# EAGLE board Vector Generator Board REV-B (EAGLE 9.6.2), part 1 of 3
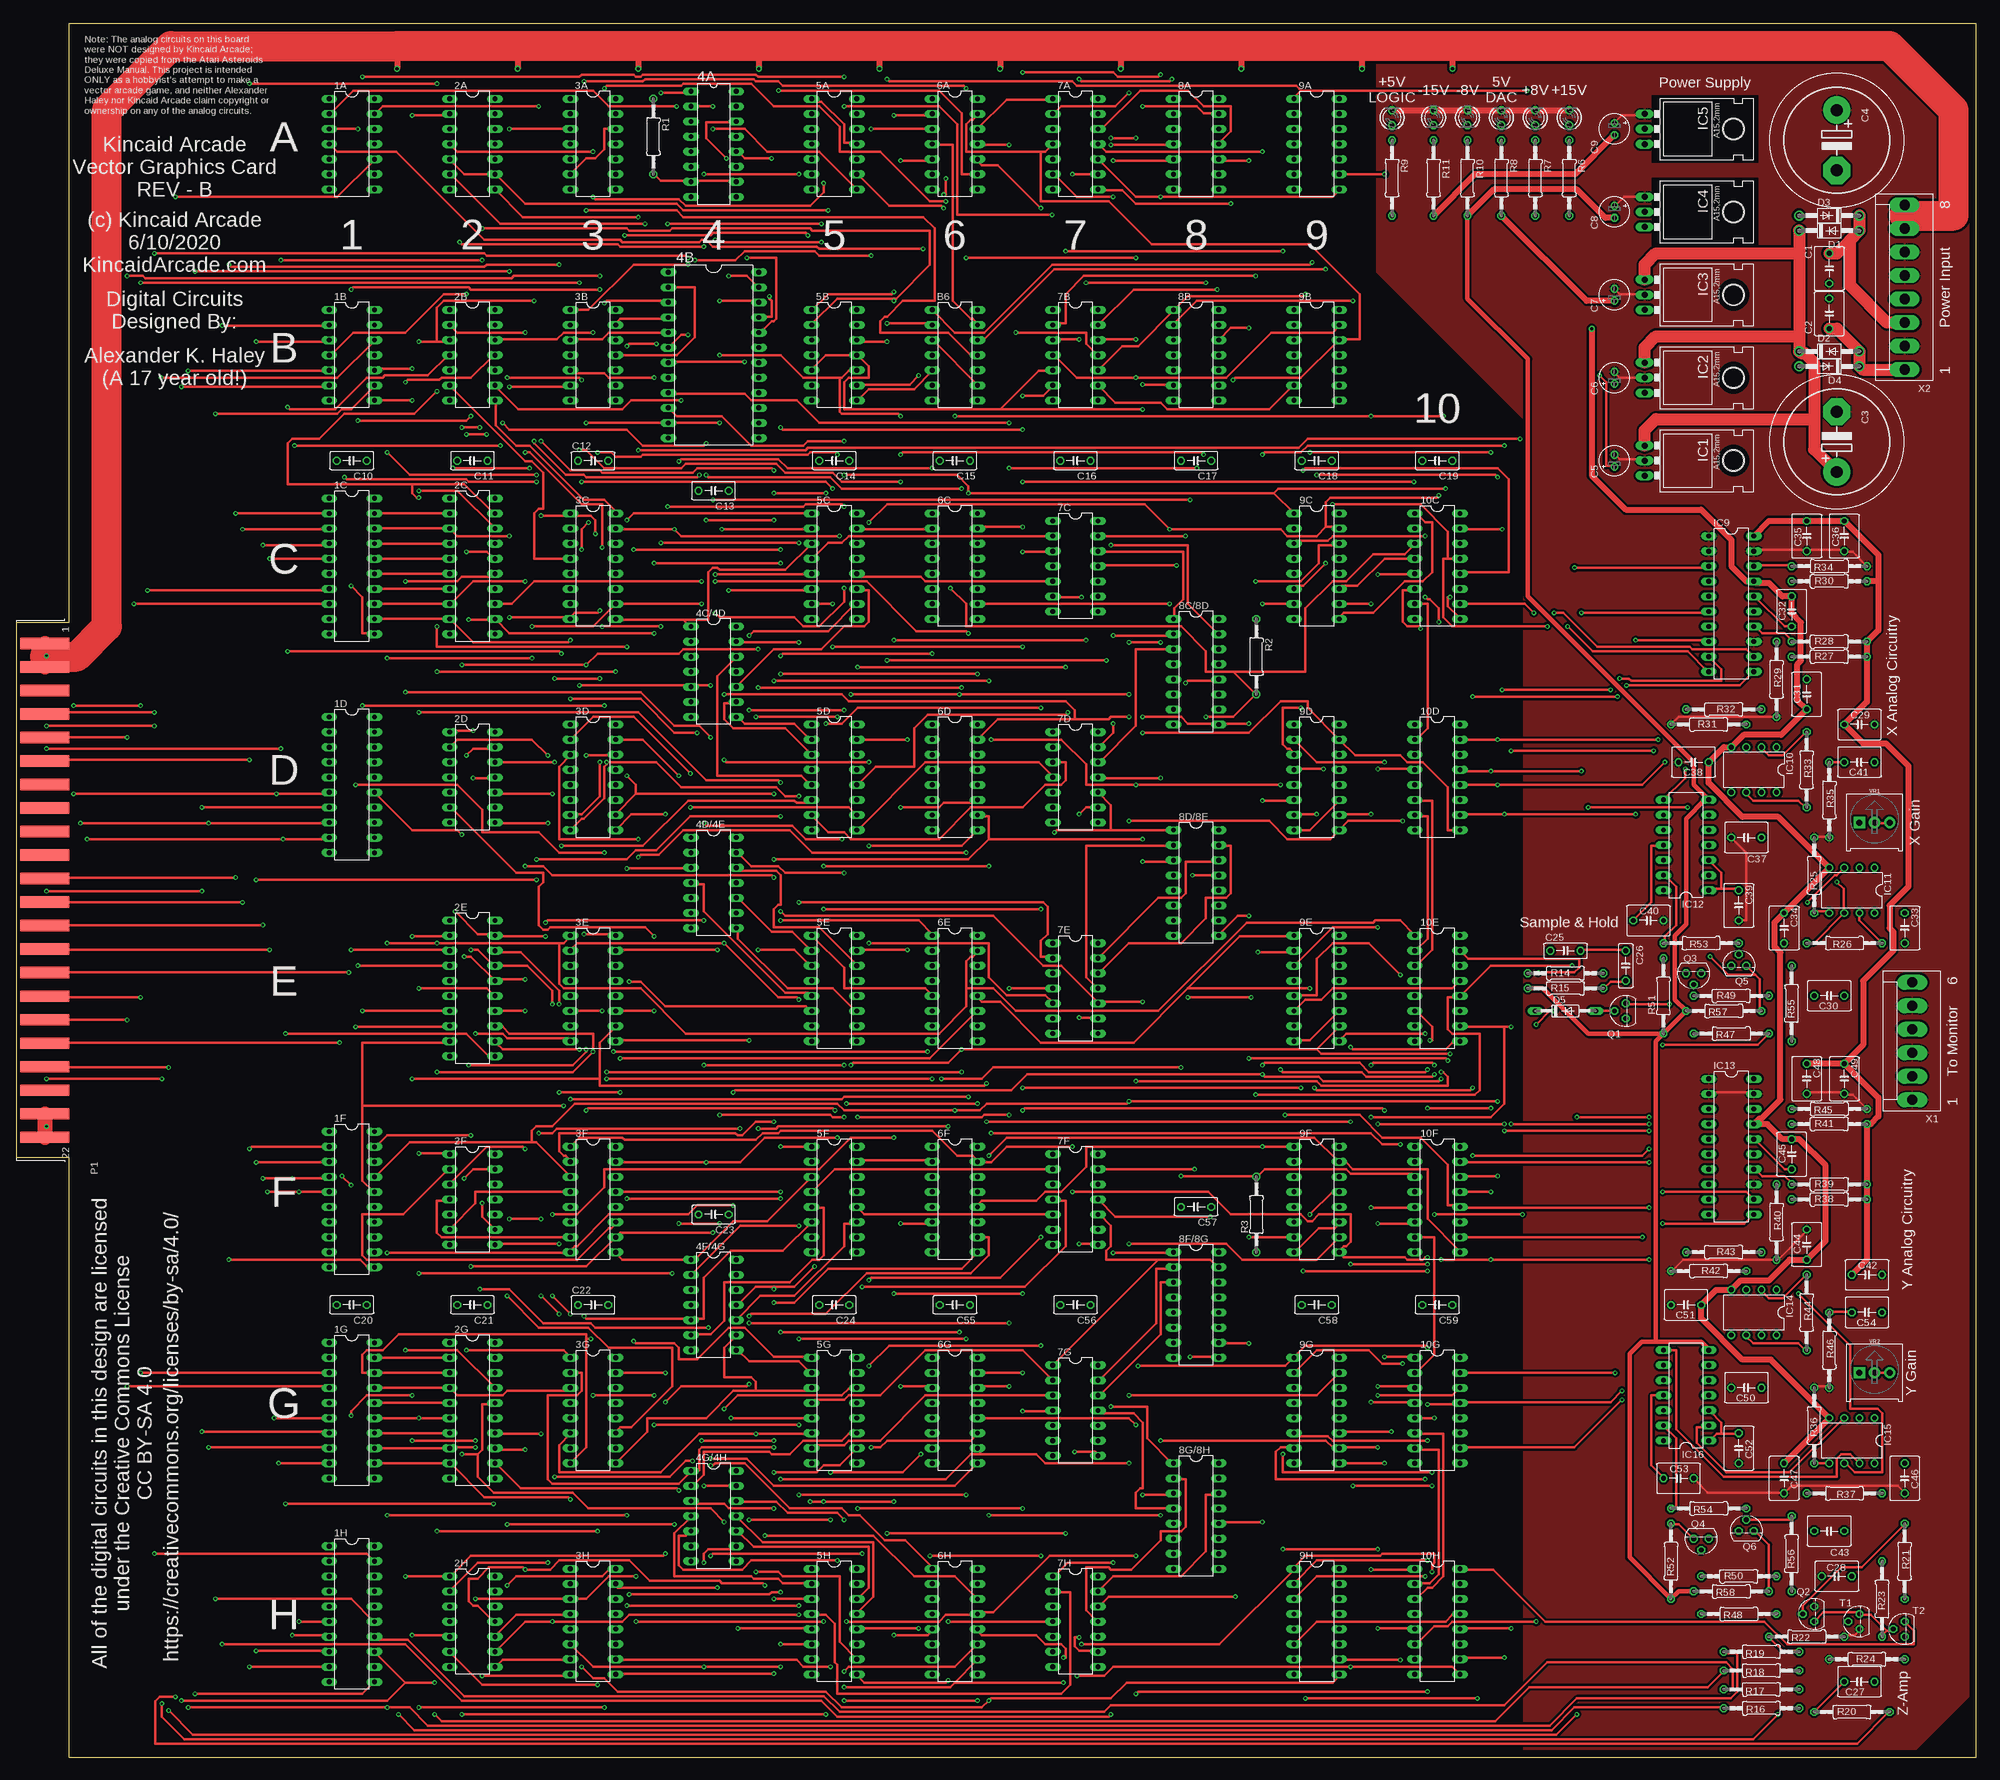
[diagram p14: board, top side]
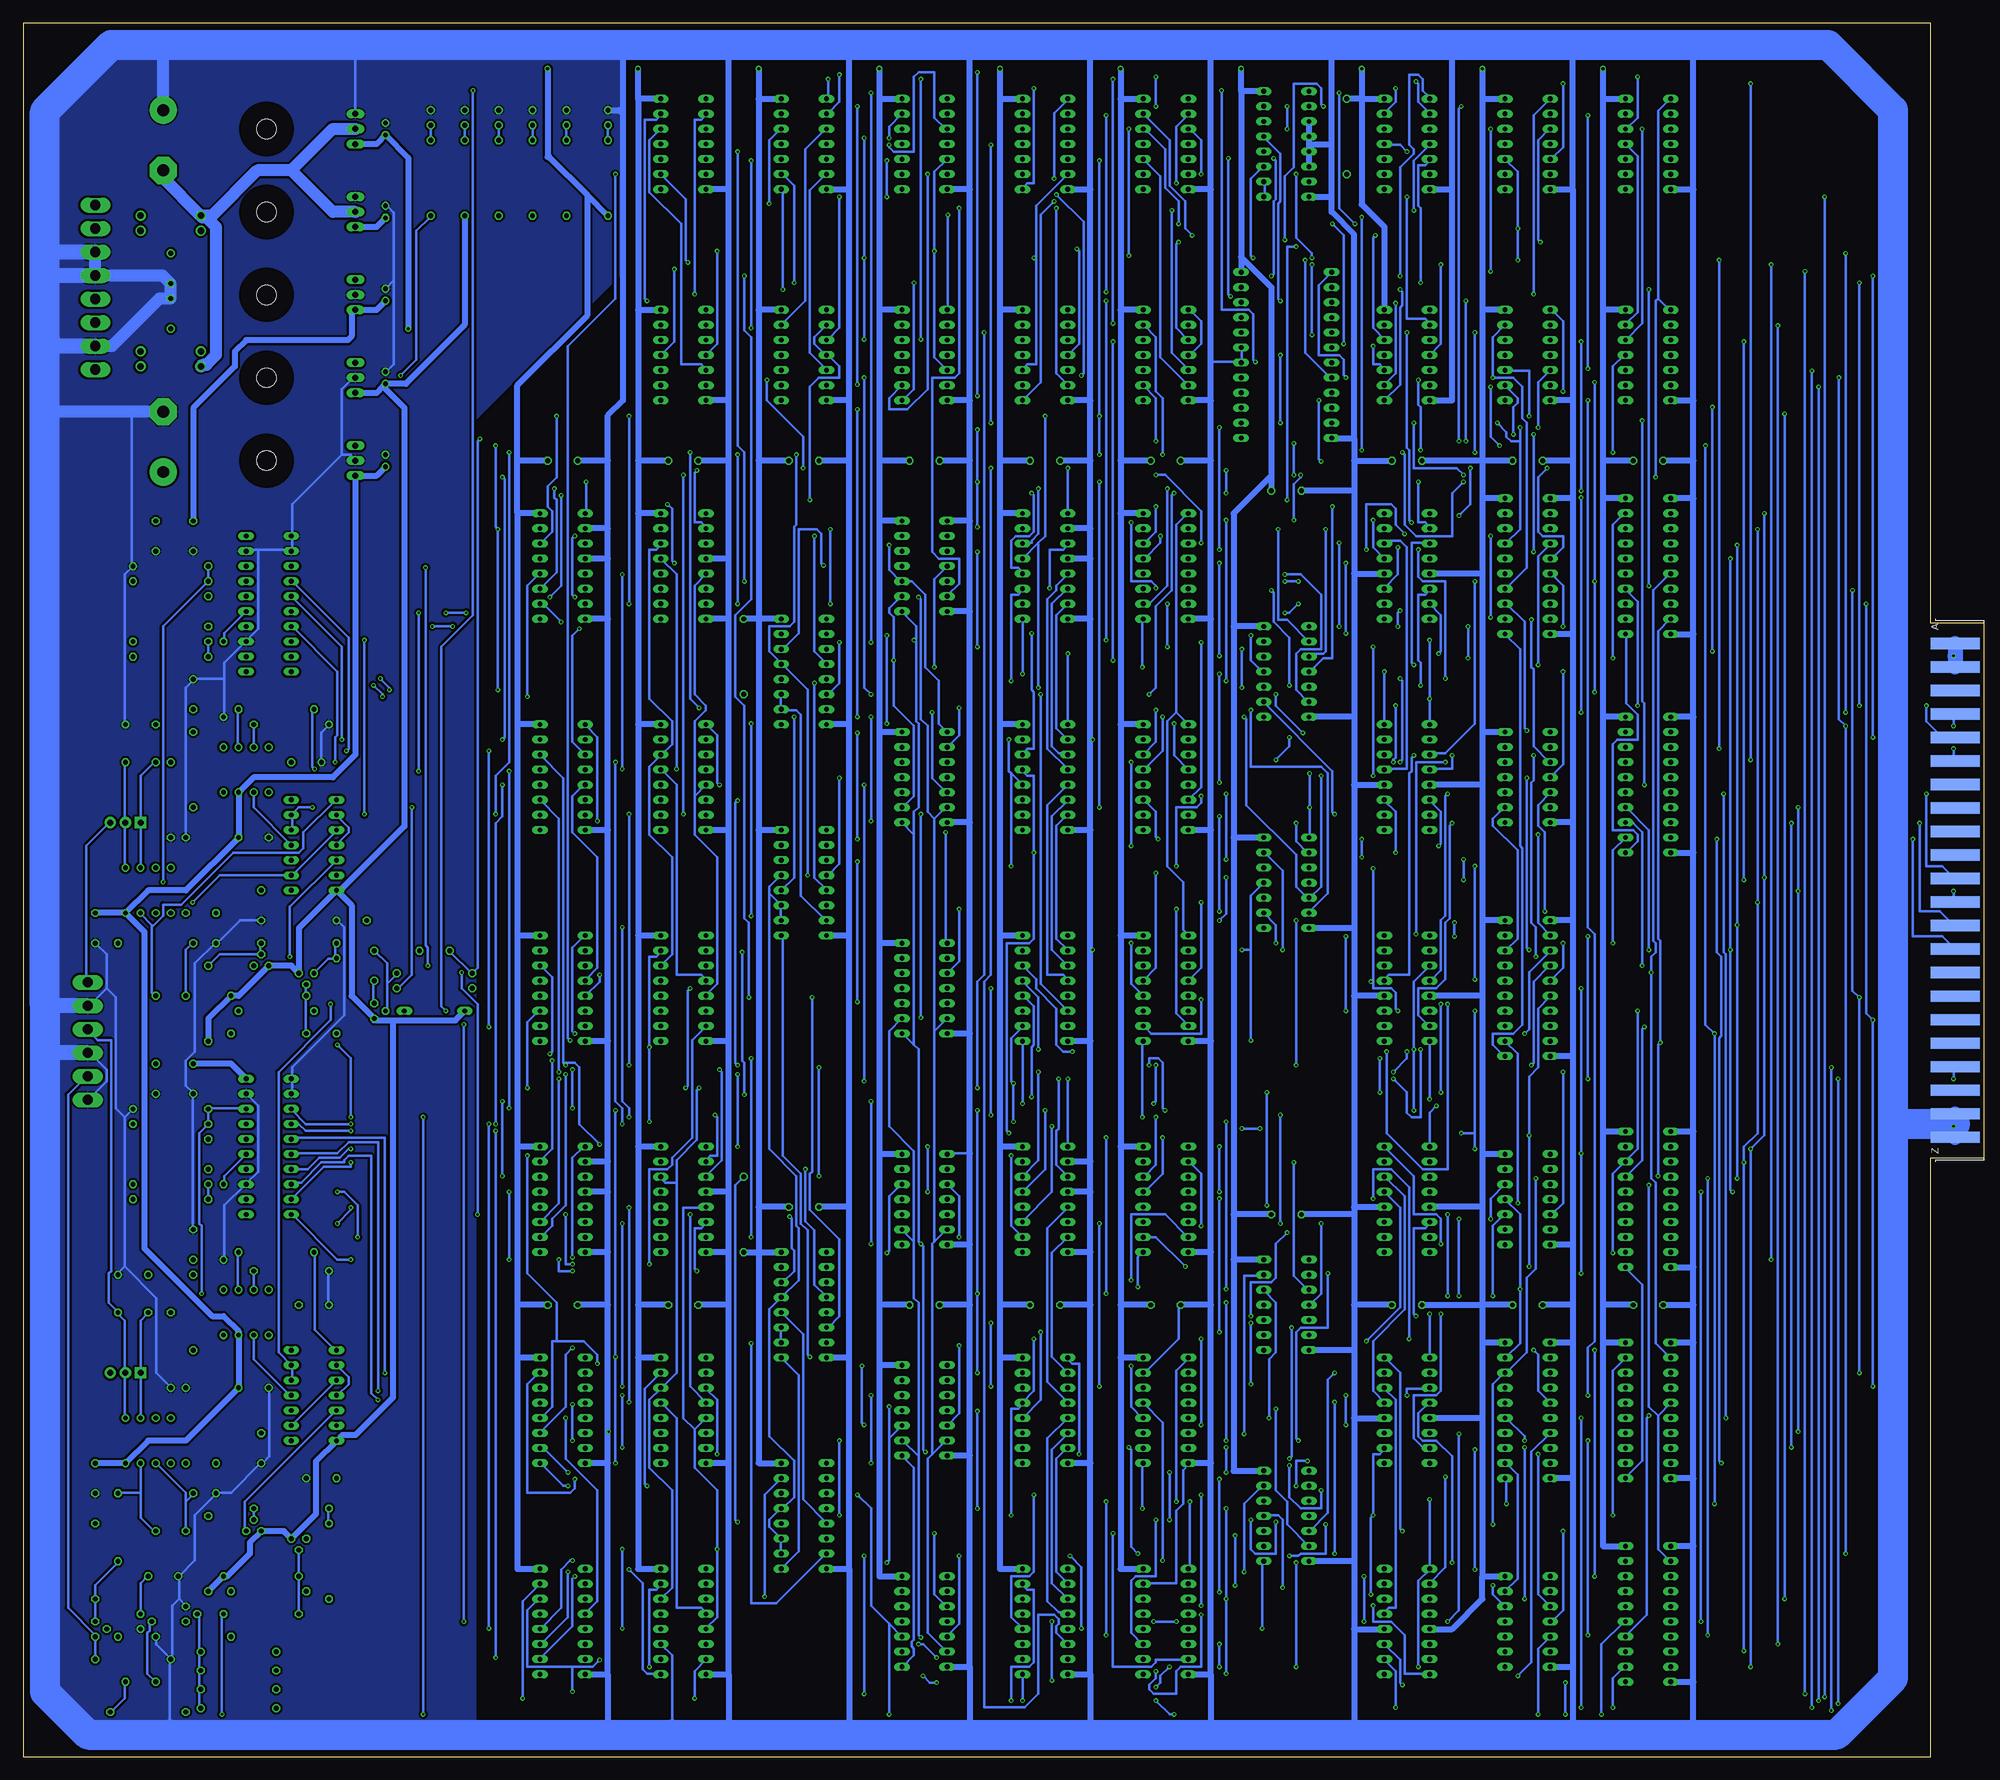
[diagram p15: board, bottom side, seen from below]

Size 330.2 x 292.1 mm. Coordinates in mm from the lower left corner, seen from the top.
Outline: 8.89,0 8.89,100.97 0,100.97 0,191.13 8.89,191.13 8.89,292.1 330.2,292.1 330.2,0 8.89,0
Copper layers (1*16): Top 0.035mm / dielectric 1.5mm / Bottom 0.035mm
Design rules "default": minimum track width 6mil, minimum drill 0.35mm, track to track 6mil, track to pad 6mil, pad to pad 6mil, via to via 6mil, smd to smd 6mil, copper to edge 40mil, drill to drill 6mil, minimum pad ring 10mil, minimum via ring 8mil, stop-mask expansion 4mil, vias tented up to drill 0mil, thermal gap 10mil
Net classes: 0 default: width 0.381 mm, clearance 0.381 mm

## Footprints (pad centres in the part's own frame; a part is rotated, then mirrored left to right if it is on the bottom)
DIL14 = drill 0.813 long: 1 -7.62,-3.81; 2 -5.08,-3.81; 3 -2.54,-3.81; 4 0,-3.81; 5 2.54,-3.81; 6 5.08,-3.81; 7 7.62,-3.81; 8 7.62,3.81; 9 5.08,3.81; 10 2.54,3.81; 11 0,3.81; 12 -2.54,3.81; 13 -5.08,3.81; 14 -7.62,3.81
DIL20 = drill 0.813 long: 1 -11.43,-3.81; 2 -8.89,-3.81; 3 -6.35,-3.81; 4 -3.81,-3.81; 5 -1.27,-3.81; 6 1.27,-3.81; 7 3.81,-3.81; 8 6.35,-3.81; 9 8.89,-3.81; 10 11.43,-3.81; 11 11.43,3.81; 12 8.89,3.81; 13 6.35,3.81; 14 3.81,3.81; 15 1.27,3.81; 16 -1.27,3.81; 17 -3.81,3.81; 18 -6.35,3.81; 19 -8.89,3.81; 20 -11.43,3.81
DIL16 = drill 0.813 long: 1 -8.89,-3.81; 2 -6.35,-3.81; 3 -3.81,-3.81; 4 -1.27,-3.81; 5 1.27,-3.81; 6 3.81,-3.81; 7 6.35,-3.81; 8 8.89,-3.81; 9 8.89,3.81; 10 6.35,3.81; 11 3.81,3.81; 12 1.27,3.81; 13 -1.27,3.81; 14 -3.81,3.81; 15 -6.35,3.81; 16 -8.89,3.81
DIL24-6 = drill 0.813 long: 1 -13.97,-7.62; 2 -11.43,-7.62; 3 -8.89,-7.62; 4 -6.35,-7.62; 5 -3.81,-7.62; 6 -1.27,-7.62; 7 1.27,-7.62; 8 3.81,-7.62; 9 6.35,-7.62; 10 8.89,-7.62; 11 11.43,-7.62; 12 13.97,-7.62; 13 13.97,7.62; 14 11.43,7.62; 15 8.89,7.62; 16 6.35,7.62; 17 3.81,7.62; 18 1.27,7.62; 19 -1.27,7.62; 20 -3.81,7.62; 21 -6.35,7.62; 22 -8.89,7.62; 23 -11.43,7.62; 24 -13.97,7.62
C050-050X075 = drill 0.813 octagon: 1 -2.54,0; 2 2.54,0
EB22,5D = drill 2.007 pad 4.597: + -5.08,0 | drill 2.007 pad 4.597 octagon: - 5.08,0
E2-5 = drill 0.813 pad 1.27: + -1.016,0 | drill 0.813 pad 1.27 octagon: - 1.016,0
C050-030X075 = drill 0.813 octagon: 1 -2.54,0; 2 2.54,0
C050-025X075 = drill 0.813 octagon: 1 -2.54,0; 2 2.54,0
DO41-10 = drill 1.118: A 5.08,0; C -5.08,0
DO35-10 = drill 0.813 long: A 5.08,0; C -5.08,0
78XXL = drill 1.016 long: GND 0,-3.81; IN -2.54,-3.81; OUT 2.54,-3.81 | hole 3.302: 0,11.176
79XXL = drill 1.016 long: GND -2.54,-3.81; IN 0,-3.81; OUT 2.54,-3.81 | hole 3.302: 0,11.176
DIL08 = drill 0.813 pad 1.27: 1 -3.81,-3.81; 2 -1.27,-3.81; 3 1.27,-3.81; 4 3.81,-3.81; 5 3.81,3.81; 6 1.27,3.81; 7 -1.27,3.81; 8 -3.81,3.81
LED3MM = drill 0.813 octagon: A -1.27,0; K 1.27,0
44PINEDGE = smd 1.905 x 8.255: 1 -41.605,4.826; 2 -37.643,4.826; 3 -33.68,4.826; 4 -29.718,4.826; 5 -25.756,4.826; 6 -21.793,4.826; 7 -17.831,4.826; 8 -13.868,4.826; 9 -9.906,4.826; 10 -5.944,4.826; 11 -1.981,4.826; 12 1.981,4.826; 13 5.944,4.826; 14 9.906,4.826; 15 13.868,4.826; 16 17.831,4.826; 17 21.793,4.826; 18 25.756,4.826; 19 29.718,4.826; 20 33.68,4.826; 21 37.643,4.826; 22 41.605,4.826 | smd 1.905 x 8.255 bottom: A -41.605,4.826; B -37.643,4.826; C -33.68,4.826; D -29.718,4.826; E -25.756,4.826; F -21.793,4.826; H -17.831,4.826; J -13.868,4.826; K -9.906,4.826; L -5.944,4.826; M -1.981,4.826; N 1.981,4.826; P 5.944,4.826; R 9.906,4.826; S 13.868,4.826; T 17.831,4.826; U 21.793,4.826; V 25.756,4.826; W 29.718,4.826; X 33.68,4.826; Y 37.643,4.826; Z 41.605,4.826
TO92 = drill 0.813 octagon: 1 1.27,0; 2 0,1.905; 3 -1.27,0
0207/12 = drill 0.813 octagon: 1 -6.35,0; 2 6.35,0
TRIMPOT-PTH-3386U = drill 1.016 pad 1.88 square: 1 -2.54,-0.015 | drill 1.016 pad 1.88: 2 0,-0.015; 3 2.54,-0.015
KK-156-6 = drill 1.7 pad 2.184 long: 1 -9.9,0; 2 -5.94,0; 3 -1.98,0; 4 1.98,0; 5 5.94,0; 6 9.9,0
KK-156-8 = drill 1.7 pad 2.184 long: 1 -13.86,0; 2 -9.9,0; 3 -5.94,0; 4 -1.98,0; 5 1.98,0; 6 5.94,0; 7 9.9,0; 8 13.86,0

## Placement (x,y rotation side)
1A  7404N  [DIL14]  56.52,271.78 270 top
1B  7402N  [DIL14]  56.52,236.22 270 top
1C  74HC573N  [DIL20]  56.52,200.66 270 top
1D  74HC573N  [DIL20]  56.52,163.83 270 top
1F  74HC573N  [DIL20]  56.52,93.98 270 top
1G  74HC573N  [DIL20]  56.52,58.42 270 top
1H  74HC573N  [DIL20]  56.52,24.13 270 top
2A  7400N  [DIL14]  76.84,271.78 270 top
2B  7404N  [DIL14]  76.84,236.22 270 top
2C  74HC573N  [DIL20]  76.84,200.66 270 top
2D  7404N  [DIL14]  76.84,165.1 270 top
2E  74HC573N  [DIL20]  76.84,129.54 270 top
2F  7404N  [DIL14]  76.84,93.98 270 top
2G  74HC573N  [DIL20]  76.84,58.42 270 top
2H  7404N  [DIL14]  76.84,22.86 270 top
3A  7432N  [DIL14]  97.16,271.78 270 top
3B  7404N  [DIL14]  97.16,236.22 270 top
3C  7483N  [DIL16]  97.16,200.66 270 top
3D  7483N  [DIL16]  97.16,165.1 270 top
3E  7483N  [DIL16]  97.16,129.54 270 top
3F  7483N  [DIL16]  97.16,93.98 270 top
3G  7483N  [DIL16]  97.16,58.42 270 top
3H  7483N  [DIL16]  97.16,22.86 270 top
4A  74161N  [DIL16]  117.48,271.78 270 top
4B  74154N  [DIL24-6]  117.48,236.22 270 top
4C/4D  7404N  [DIL14]  117.48,182.88 270 top
4D/4E  7404N  [DIL14]  117.48,147.32 270 top
4F/4G  7404N  [DIL14]  117.48,76.2 270 top
4G/4H  7404N  [DIL14]  117.48,40.64 270 top
5A  7432N  [DIL14]  137.8,271.78 270 top
5B  74S11N  [DIL14]  137.8,236.22 270 top
5C  74157N  [DIL16]  137.8,200.66 270 top
5D  74157N  [DIL16]  137.8,165.1 270 top
5E  74157N  [DIL16]  137.8,129.54 270 top
5F  74157N  [DIL16]  137.8,93.98 270 top
5G  74157N  [DIL16]  137.8,58.42 270 top
5H  74157N  [DIL16]  137.8,22.86 270 top
6A  7404N  [DIL14]  158.12,271.78 270 top
6C  7485N  [DIL16]  158.12,200.66 270 top
6D  7485N  [DIL16]  158.12,165.1 270 top
6E  7485N  [DIL16]  158.12,129.54 270 top
6F  7485N  [DIL16]  158.12,93.98 270 top
6G  7485N  [DIL16]  158.12,58.42 270 top
6H  7485N  [DIL16]  158.12,22.86 270 top
7A  74S08N  [DIL14]  178.44,271.78 270 top
7B  74S08N  [DIL14]  178.44,236.22 270 top
7C  7495N  [DIL14]  178.44,200.66 270 top
7D  7495N  [DIL14]  178.44,165.1 270 top
7E  7495N  [DIL14]  178.44,129.54 270 top
7F  7495N  [DIL14]  178.44,93.98 270 top
7G  7495N  [DIL14]  178.44,58.42 270 top
7H  7495N  [DIL14]  178.44,22.86 270 top
8A  7432N  [DIL14]  198.75,271.78 270 top
8B  74S11N  [DIL14]  198.75,236.22 270 top
8C/8D  7497N  [DIL16]  198.75,182.88 270 top
8D/8E  7497N  [DIL16]  198.75,147.32 270 top
8F/8G  7497N  [DIL16]  198.75,76.2 270 top
8G/8H  7497N  [DIL16]  198.75,40.64 270 top
9A  7404N  [DIL14]  219.07,271.78 270 top
9B  74S08N  [DIL14]  219.07,236.22 270 top
9C  74191N  [DIL16]  219.07,200.66 270 top
9D  74191N  [DIL16]  219.07,165.1 270 top
9E  74191N  [DIL16]  219.07,129.54 270 top
9F  74191N  [DIL16]  219.07,93.98 270 top
9G  74191N  [DIL16]  219.07,58.42 270 top
9H  74191N  [DIL16]  219.07,22.86 270 top
10C  7485N  [DIL16]  239.4,200.66 270 top
10D  7485N  [DIL16]  239.4,165.1 270 top
10E  7485N  [DIL16]  239.4,129.54 270 top
10F  7485N  [DIL16]  239.4,93.98 270 top
10G  7485N  [DIL16]  239.4,58.42 270 top
10H  7485N  [DIL16]  239.4,22.86 270 top
B6  74S08N  [DIL14]  158.12,236.22 270 top
C1  .1 uf  [C050-050X075]  305.44,250.82 270 top
C2  .1 uf  [C050-050X075]  305.44,243.21 90 top
C3  470 uf  [EB22,5D]  306.71,221.62 90 top
C4  470 uf  [EB22,5D]  306.71,272.41 270 top
C5  1 uf  [E2-5]  269.24,218.44 90 top
C6  1uf  [E2-5]  269.24,232.41 90 top
C7  1 uf  [E2-5]  269.24,246.38 90 top
C8  1uf  [E2-5]  269.24,260.35 270 top
C9  1 uf  [E2-5]  269.24,274.32 270 top
C10  .1uf  [C050-030X075]  56.52,218.44 180 top
C11  .1uf  [C050-030X075]  76.84,218.44 180 top
C12  .1uf  [C050-030X075]  97.16,218.44 0 top
C13  .1uf  [C050-030X075]  117.48,213.36 180 top
C14  .1uf  [C050-030X075]  137.8,218.44 180 top
C15  .1uf  [C050-030X075]  158.12,218.44 180 top
C16  .1uf  [C050-030X075]  178.44,218.44 180 top
C17  .1uf  [C050-030X075]  198.75,218.44 180 top
C18  .1uf  [C050-030X075]  219.07,218.44 180 top
C19  .1uf  [C050-030X075]  239.4,218.44 180 top
C20  .1uf  [C050-030X075]  56.52,76.2 180 top
C21  .1uf  [C050-030X075]  76.84,76.2 180 top
C22  .1uf  [C050-030X075]  97.16,76.2 0 top
C23  .1uf  [C050-030X075]  117.48,91.44 180 top
C24  .1uf  [C050-030X075]  137.8,76.2 180 top
C25  390pf  [C050-025X075]  260.99,135.89 0 top
C26  100pf  [C050-025X075]  271.14,133.35 270 top
C27  270pf  [C050-050X075]  310.51,12.7 180 top
C28  .01uf  [C050-050X075]  306.71,30.48 180 top
C29  .1uf  [C050-050X075]  310.51,173.99 0 top
C30  10pf  [C050-050X075]  305.44,128.27 180 top
C31  .1uf  [C050-050X075]  301.62,179.07 90 top
C32  .01uf  [C050-050X075]  299.09,193.04 90 top
C33  .1uf  [C050-050X075]  318.13,139.7 270 top
C34  .1uf  [C050-050X075]  297.81,139.7 270 top
C35  .1uf  [C050-050X075]  301.62,205.74 270 top
C36  .1uf  [C050-050X075]  307.98,205.74 270 top
C37  .1uf  [C050-050X075]  291.47,154.94 180 top
C38  .1uf  [C050-050X075]  282.58,167.64 180 top
C39  220pf  [C050-050X075]  290.19,143.51 270 top
C40  220pf  [C050-050X075]  274.96,140.97 0 top
C41  69pf  [C050-050X075]  310.51,167.64 180 top
C42  .1uf  [C050-050X075]  311.78,81.28 0 top
C43  10pf  [C050-050X075]  305.44,38.1 180 top
C44  .1uf  [C050-050X075]  301.62,86.36 90 top
C45  .01uf  [C050-050X075]  299.09,101.6 90 top
C46  .1uf  [C050-050X075]  318.13,46.99 270 top
C47  .1uf  [C050-050X075]  297.81,46.99 270 top
C48  .1uf  [C050-050X075]  301.62,114.3 270 top
C49  .1uf  [C050-050X075]  307.98,114.3 270 top
C50  .1uf  [C050-050X075]  291.47,62.23 180 top
C51  .1uf  [C050-050X075]  281.31,76.2 180 top
C52  220pf  [C050-050X075]  290.19,52.07 270 top
C53  220pf  [C050-050X075]  280.03,46.99 0 top
C54  69pf  [C050-050X075]  311.78,74.93 180 top
C55  .1uf  [C050-030X075]  158.12,76.2 180 top
C56  .1uf  [C050-030X075]  178.44,76.2 180 top
C57  .1uf  [C050-030X075]  198.75,92.71 180 top
C58  .1uf  [C050-030X075]  219.07,76.2 180 top
C59  .1uf  [C050-030X075]  239.4,76.2 180 top
D1  1N4004  [DO41-10]  305.44,257.18 0 top
D2  1N4004  [DO41-10]  305.44,236.85 0 top
D3  1N4004  [DO41-10]  305.44,259.72 180 top
D4  1N4004  [DO41-10]  305.44,234.31 180 top
D5  1N4148  [DO35-10]  260.99,125.73 0 top
IC1  7815  [78XXL]  278.13,218.44 270 top
IC2  7808  [78XXL]  278.13,232.41 270 top
IC3  7805  [78XXL]  278.13,246.38 270 top
IC4  7908  [79XXL]  278.13,260.35 270 top
IC5  7915  [79XXL]  278.13,274.32 270 top
IC9  DAC312  [DIL20]  288.93,194.31 270 top
IC10  TL081P  [DIL08]  292.74,166.37 180 top
IC11  TL082P  [DIL08]  309.25,146.05 180 top
IC12  4016N  [DIL14]  281.31,153.67 90 top
IC13  DAC312  [DIL20]  288.93,102.87 270 top
IC14  TL081P  [DIL08]  292.74,74.93 180 top
IC15  TL082P  [DIL08]  309.25,53.34 180 top
IC16  4016N  [DIL14]  281.31,60.96 90 top
LED1  [LED3MM]  261.62,276.23 90 top
LED2  [LED3MM]  255.91,276.23 90 top
LED3  [LED3MM]  250.19,276.23 90 top
LED4  [LED3MM]  231.78,276.23 90 top
LED5  [LED3MM]  244.47,276.23 270 top
LED6  [LED3MM]  238.76,276.23 270 top
P1  44PINEDGE  [44PINEDGE]  0,146.05 270 top
Q1  2N3906  [TO92]  271.14,125.73 90 top
Q2  2N3906  [TO92]  302.89,24.13 90 top
Q3  2N3906  [TO92]  282.58,132.08 180 top
Q4  2N3906  [TO92]  283.85,36.83 180 top
Q5  2N3906  [TO92]  290.19,133.35 0 top
Q6  2N3906  [TO92]  291.47,38.1 0 top
R1  1K  [0207/12]  107.32,273.05 270 top
R2  1K  [0207/12]  208.92,185.42 270 top
R3  1K  [0207/12]  208.92,91.44 90 top
R6  680  [0207/12]  261.62,266.06 270 top
R7  330  [0207/12]  255.91,266.06 270 top
R8  150  [0207/12]  250.19,266.06 270 top
R9  150  [0207/12]  231.78,266.06 270 top
R10  330  [0207/12]  244.47,266.06 270 top
R11  680  [0207/12]  238.76,266.06 270 top
R14  47K  [0207/12]  260.99,132.08 0 top
R15  330  [0207/12]  260.99,129.54 0 top
R16  1.2K  [0207/12]  294,8.26 0 top
R17  2.2K  [0207/12]  294,11.43 0 top
R18  4.7K  [0207/12]  294,14.61 0 top
R19  10K  [0207/12]  294,17.78 0 top
R20  1K  [0207/12]  309.25,7.62 0 top
R21  3.9K  [0207/12]  318.13,33.02 270 top
R22  22K  [0207/12]  301.62,20.32 180 top
R23  68  [0207/12]  314.33,26.67 90 top
R24  27  [0207/12]  311.78,16.51 0 top
R25  6.8K  [0207/12]  302.89,148.59 270 top
R26  8.2K  [0207/12]  307.98,137.16 180 top
R27  10k  [0207/12]  305.44,185.42 0 top
R28  10k  [0207/12]  305.44,187.96 0 top
R29  4.7K  [0207/12]  296.55,181.61 270 top
R30  10K  [0207/12]  305.44,198.12 0 top
R31  4.7K  [0207/12]  285.12,173.99 0 top
R32  10K  [0207/12]  287.65,176.53 0 top
R33  10K  [0207/12]  301.62,166.37 270 top
R34  2.2K  [0207/12]  305.44,200.66 180 top
R35  3.9K  [0207/12]  305.44,161.29 270 top
R36  6.8K  [0207/12]  302.89,55.88 270 top
R37  8.2K  [0207/12]  307.98,44.45 180 top
R38  10k  [0207/12]  305.44,93.98 0 top
R39  10k  [0207/12]  305.44,96.52 0 top
R40  4.7K  [0207/12]  296.55,90.17 270 top
R41  10K  [0207/12]  305.44,106.68 0 top
R42  4.7K  [0207/12]  285.12,81.91 0 top
R43  10K  [0207/12]  287.65,85.09 0 top
R44  10K  [0207/12]  301.62,74.93 270 top
R45  2.2K  [0207/12]  305.44,109.22 180 top
R46  3.9K  [0207/12]  305.44,68.58 270 top
R47  18K  [0207/12]  288.93,121.92 180 top
R48  18K  [0207/12]  290.19,24.13 180 top
R49  2.2K  [0207/12]  288.93,128.27 0 top
R50  2.2K  [0207/12]  290.19,30.48 0 top
R51  3.3K  [0207/12]  277.5,128.27 90 top
R52  3.3K  [0207/12]  278.76,33.02 90 top
R53  100K  [0207/12]  283.85,137.16 180 top
R54  100K  [0207/12]  285.12,41.91 180 top
R55  4.7K  [0207/12]  299.09,127 90 top
R56  4.7K  [0207/12]  299.09,34.29 90 top
R57  56K  [0207/12]  287.65,125.73 180 top
R58  56K  [0207/12]  288.93,27.94 180 top
T1  2N3904  [TO92]  310.51,22.86 90 top
T2  2N3904  [TO92]  318.13,21.59 90 top
VR1  10k  [TRIMPOT-PTH-3386U]  313.06,157.48 0 top
VR2  10k  [TRIMPOT-PTH-3386U]  313.06,64.77 0 top
X1  [KK-156-6]  319.4,120.65 90 top
X2  [KK-156-8]  318.13,247.65 90 top

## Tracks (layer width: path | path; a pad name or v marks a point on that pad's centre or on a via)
1DX0
  Top 0.381: 112.4,191.64 113.54,190.5 4C/4D.1 | 112.4,191.64 100.97,191.64 3C.9 | 5C.3 129.54,200.03 118.49,200.03 118.11,200.41 117.35,200.41 116.59,199.64 116.59,191.64 112.4,191.64
1DX1  (via drill 0.35)
  Top 0.381: v94.87,180.59 113.54,180.59 4C/4D.5 113.92,180.59 v116.97,180.59 | v120.02,196.6 133.73,196.6 5C.6
  Bottom 0.381: v94.87,180.59 94.87,184.4 95.25,184.78 95.25,195.83 94.11,195.83 93.34,196.6 3C.6 | v120.02,196.6 119.63,196.22 119.63,191.26 116.97,188.59 v116.97,180.59
1DX2  (via drill 0.35)
  Top 0.381: v95.25,214.88 136.4,214.88 v137.54,213.74 | v123.44,188.98 124.21,189.74 136.78,189.74 141.35,194.31 5C.10
  Bottom 0.381: v95.25,214.88 95.25,208.03 94.11,208.03 93.34,207.26 3C.2 | v137.54,213.74 137.54,197.36 140.59,194.31 5C.10 | v123.44,188.98 123.44,184.78 121.54,182.88 4C/4D.11
1DX3  (via drill 0.35)
  Top 0.381: 3C.15 100.97,206.88 v110.87,206.88 112.01,205.74 v138.68,205.74
  Bottom 0.381: v110.87,206.88 110.87,186.31 111.25,185.93 113.54,185.93 113.54,185.55 4C/4D.3 | v138.68,205.74 138.68,204.6 141.35,201.93 5C.13
1DX4  (via drill 0.35)
  Top 0.381: 3D.9 103.63,158.88 v109.35,158.88 | 5D.3 129.54,173.36 120.78,173.36 119.25,174.88 119.25,177.55 121.16,177.55 4C/4D.9
  Bottom 0.381: v109.35,158.88 109.73,159.26 109.73,166.12 121.16,177.55 4C/4D.9
1DX5  (via drill 0.35)
  Top 0.381: v91.82,153.54 105.54,153.54 113.16,161.16 131.06,161.16 131.44,160.78 133.35,160.78 133.73,161.16 5D.6 | v131.83,187.83 121.54,187.83 4C/4D.13
  Bottom 0.381: v91.82,153.54 91.44,153.92 91.44,159.26 93.34,161.16 3D.6 | v131.83,187.83 131.83,163.45 5D.6
1DX6  (via drill 0.35)
  Top 0.381: 3D.2 97.16,175.26 104.01,175.26 v113.54,165.74 | v113.54,160.02 140.21,160.02 141.35,158.88 5D.10
  Bottom 0.381: v113.54,165.74 v113.54,160.02 113.54,155.07 4D/4E.1
1DX7  (via drill 0.35)
  Top 0.381: v111.63,165.35 105.54,171.45 3D.15 | v124.59,175.26 v138.3,175.26
  Bottom 0.381: v111.63,165.35 111.63,146.69 113.54,144.78 4D/4E.5 113.92,144.78 115.82,146.69 115.82,152.02 124.21,160.4 124.21,174.88 v124.59,175.26 | v138.3,175.26 138.3,169.55 141.35,166.5 5D.13
1DX8  (via drill 0.35)
  Top 0.381: v123.44,120.78 100.97,120.78 3E.9 | v124.97,136.02 131.06,136.02 133.73,133.35 5E.3
  Bottom 0.381: 123.44,136.02 123.44,145.16 4D/4E.11 | 123.44,136.02 v123.44,120.78 | 123.44,136.02 v124.97,136.02
1DX9  (via drill 0.35)
  Top 0.381: v98.68,125.73 3E.6 | v102.87,149.73 113.54,149.73 4D/4E.3 | v103.25,130.68 105.16,130.68 109.35,126.49 132.97,126.49 133.73,125.73 5E.6
  Bottom 0.381: v98.68,125.73 99.06,126.11 99.06,128.78 99.82,129.54 102.87,129.54 102.87,130.68 | v102.87,149.73 102.87,130.68 | 102.87,130.68 v103.25,130.68
1DX10  (via drill 0.35)
  Top 0.381: 3E.2 93.34,136.02 94.49,137.16 v119.25,137.16 128.4,128.02 131.44,128.02 v131.83,127.64
  Bottom 0.381: v119.25,137.16 119.25,140.21 4D/4E.9 | v131.83,127.64 131.83,121.92 140.21,121.92 141.35,123.06 5E.10
1DX11  (via drill 0.35)
  Top 0.381: v118.11,136.02 100.97,136.02 3E.15 | v139.45,148.97 129.54,148.97 128.4,150.11 123.83,150.11 121.54,152.4 4D/4E.13
  Bottom 0.381: v118.11,136.02 118.11,149.35 121.16,152.4 4D/4E.13 | 5E.13 139.45,132.97 v139.45,148.97
1DY0
  Top 0.381: 3F.9 100.97,84.96 102.11,83.82 4F/4G.1 114.3,83.82 120.78,90.3 126.49,90.3 5F.3
1DY1  (via drill 0.35)
  Top 0.381: v95.63,74.3 96.01,73.91 113.54,73.91 4F/4G.5 113.92,73.91 115.82,73.91 115.82,80.77 120.4,85.34 129.16,85.34 5F.6
  Bottom 0.381: v95.63,74.3 96.01,74.68 96.01,89.15 94.11,89.15 93.34,89.92 3F.6
1DY2  (via drill 0.35)
  Top 0.381: 127.64,79.25 131.06,79.25 v134.49,82.68 | 127.64,79.25 124.59,79.25 121.54,76.2 4F/4G.11 | v127.64,107.06 124.59,107.06 122.3,104.78 121.54,104.78 121.16,105.16 91.44,105.16 91.44,102.11 92.2,101.35 92.58,101.35 93.34,100.58 3F.2 | 127.64,79.25 v127.64,78.87
  Bottom 0.381: v134.49,82.68 139.45,87.63 5F.10 | v127.64,78.87 v127.64,107.06
1DY3  (via drill 0.35)
  Top 0.381: 3F.15 100.97,100.2 v116.21,100.2 121.92,100.2 126.11,104.39 v138.3,104.39
  Bottom 0.381: v116.21,100.2 116.21,81.15 113.92,78.87 4F/4G.3 | v138.3,104.39 138.3,98.3 141.35,95.25 5F.13
1DY4
  Top 0.381: 3G.9 106.3,54.86 106.3,57.15 116.21,57.15 120.78,61.72 124.59,61.72 | 124.59,61.72 133.35,61.72 133.73,62.1 5G.3 | 124.59,61.72 124.59,63.25 123.83,64.01 119.25,64.01 119.25,68.96 121.16,70.87 4F/4G.9
1DY5  (via drill 0.35)
  Top 0.381: 3G.6 93.34,54.48 91.44,52.58 91.44,48.01 108.59,48.01 115.06,54.48 v124.59,54.48 133.73,54.48 5G.6
  Bottom 0.381: v124.59,54.48 124.59,81.15 121.54,81.15 4F/4G.13
1DY6  (via drill 0.35)
  Top 0.381: 3G.2 95.25,64.77 95.25,61.72 94.49,60.96 89.54,60.96 89.54,46.86 90.3,46.1 111.63,46.1 113.54,48.01 4G/4H.1 113.92,48.39 115.06,48.39 115.06,51.82 115.44,52.2 v127.64,52.2 | 5G.10 138.68,49.15 136.02,49.15 134.87,48.01 v127.64,48.01
  Bottom 0.381: v127.64,52.2 v127.64,48.01
1DY7  (via drill 0.35)
  Top 0.381: v109.35,64.77 3G.15 | v138.3,33.15 123.83,33.15 122.3,31.62 112.4,31.62 111.63,32.39 111.63,37.34 112.78,37.34 113.54,38.1 4G/4H.5
  Bottom 0.381: v109.35,64.77 110.49,63.63 110.49,41.15 113.54,38.1 4G/4H.5 | 5G.13 138.3,56.39 v138.3,33.15
1DY8  (via drill 0.35)
  Top 0.381: v127.64,14.1 100.97,14.1 3H.9 | 5H.3 v127.64,26.67 | v127.64,41.91 120.02,41.91 119.25,42.67 114.3,42.67 113.92,43.05 4G/4H.3
  Bottom 0.381: v127.64,14.1 v127.64,26.67 v127.64,41.91
1DY9  (via drill 0.35)
  Top 0.381: 3H.6 97.16,15.24 v115.82,15.24 v128.78,15.24 | 5H.6 v128.78,19.05 | 4G/4H.9 120.78,35.05 116.59,35.05 115.82,34.29 v115.82,32.77
  Bottom 0.381: v128.78,19.05 v128.78,15.24 | v115.82,15.24 v115.82,32.77
1DY10  (via drill 0.35)
  Top 0.381: v90.68,47.24 110.11,47.24 112.78,49.91 v113.92,49.91 | 4G/4H.13 v115.82,45.72 | 5H.10 138.68,19.43 138.68,30.48 129.16,30.48 128.4,31.24 v124.59,31.24
  Bottom 0.381: v90.68,47.24 90.68,32 93.34,29.34 3H.2 | v113.92,49.91 115.82,49.91 v115.82,45.72 | v124.59,31.24 124.59,42.67 121.54,45.72 4G/4H.13
1DY11  (via drill 0.35)
  Top 0.381: 4G/4H.11 125.73,36.2 144.4,36.2 144.4,27.05 141.73,24.38 5H.13 | v118.11,28.58 101.35,28.58 100.97,28.96 3H.15
  Bottom 0.381: v118.11,28.58 118.11,40.01 118.87,40.77 121.16,40.77 4G/4H.11
2.5MHZ  (via drill 0.35)
  Top 0.381: v207.65,141.73 205.74,141.73 202.69,138.68 8D/8E.9 | v207.65,174.12 202.69,174.12 8C/8D.9 202.31,174.12 197.36,174.12 196.22,175.26 v189.74,175.26 | v197.74,67.44 202.31,67.44 8F/8G.9 | 2A.5 73.15,268.99 75.44,266.7 2A.9 80.77,266.7 85.73,261.75 111.25,261.75 112.4,260.6 v136.78,260.6 | 5B.5 134.11,233.93 136.4,236.22 5B.11 141.73,236.22 143.64,234.31 143.64,232.41 140.21,232.41 139.45,231.65 139.45,227.08 165.74,227.08 | v176.78,253.75 v213.36,253.75 | 165.74,227.08 172.21,233.55 174.5,233.55 7B.5 | v70.87,281.94 v39.24,281.94 | P1.6 5.08,168.02 v39.24,168.02 | 165.74,227.08 v189.74,227.08
  Bottom 0.381: 8G/8H.9 199.64,34.67 199.64,64.39 8F/8G.9 | v207.65,174.12 v207.65,141.73 | v197.74,67.44 198.12,67.82 198.12,88.77 199.26,89.92 199.26,98.3 202.31,101.35 202.31,138.3 8D/8E.9 | 7B.5 176.78,235.84 v176.78,253.75 176.78,267.08 7A.5 | 9B.4 213.36,238.12 v213.36,253.75 | v136.78,260.6 136.78,236.6 134.11,233.93 5B.5 | v39.24,281.94 v39.24,168.02 | v70.87,281.94 70.87,271.27 72.77,269.37 2A.5 | v189.74,227.08 v189.74,175.26
5MHZ  (via drill 0.35)
  Top 0.381: v179.07,86.49 182.12,86.49 7F.8 | v178.31,51.44 181.74,51.44 182.12,51.05 7G.8 | 147.83,245.75 148.21,245.75 153.92,251.46 153.92,257.18 134.11,257.18 133.73,257.56 110.49,257.56 110.11,257.18 103.25,257.18 102.87,257.56 v78.49,257.56 | 147.83,245.75 138.3,245.75 134.11,241.55 5B.2 | v78.49,252.22 v44.58,252.22 | v147.83,188.21 v180.21,188.21 | 147.83,245.75 v147.83,245.36 | v44.58,169.93 v5.08,169.93
  Bottom 0.381: 7G.8 180.21,48.77 180.21,19.81 180.59,19.43 180.59,18.67 180.21,18.29 180.21,17.15 182.12,15.24 7H.8 | 180.21,120.02 182.12,121.92 7E.8 | 180.21,120.02 179.45,119.25 179.45,86.87 v179.07,86.49 178.69,86.11 178.69,51.82 v178.31,51.44 | 180.21,155.45 7D.8 | 180.21,120.02 180.21,155.45 | 179.83,188.21 179.83,174.5 179.45,174.12 179.45,160.02 180.21,159.26 180.21,155.45 | 179.83,188.21 179.83,190.5 182.12,192.79 7C.8 | 2A.10 78.49,267.08 v78.49,257.56 v78.49,252.22 | v5.08,169.93 5.08,168.02 P1.F | v44.58,252.22 v44.58,169.93 | v180.21,188.21 179.83,188.21 | v147.83,245.36 v147.83,188.21
36VAC_A
  Top 2.032: D3.C D1.A 308.93,255.59 | C1.1 306.71,253.37 308.93,255.59 | X2.3 315.19,241.71 308.93,247.97 308.93,255.59
36VAC_B
  Top 2.032: X2.1 311.04,233.79 D4.C D2.A 306.71,240.66 C2.1
+5V_DAC
  Top 1.016: C7.+ 264.54,245.36 R8.2 | IC9.20 295.27,208.28 C35.1 C36.1 313.69,202.56 313.69,198.12 | 313.69,198.12 R30.2 | 313.69,198.12 313.69,189.87 R28.2 R27.2 311.78,177.8 C29.1 311.15,170.81 314.96,170.81 318.77,167 318.77,146.69 315.6,143.51 315.6,139.7 316.23,139.06 316.23,135.89 311.15,130.81 311.15,120.02 C49.1 | C49.1 C48.1 | C49.1 313.69,111.12 313.69,107.95 312.42,106.68 R41.2 R39.2 R38.2 311.78,83.82 C42.1
  Bottom 1.016: C7.+ 270.76,243.84 IC3.OUT 274.96,243.21 274.96,239.4 275.59,238.76 292.74,238.76 294.64,236.85 294.64,234.31 301.62,227.33 C35.1 | IC13.20 295.27,116.84 C48.1
+8VDC
  Bottom 1.016: IC2.OUT 270.76,229.87 269.69,230.95 | 269.69,230.95 C6.+ 265.81,231.39 255.91,241.3 R7.2 | 269.69,230.95 266.06,227.33 266.06,156.84 276.86,146.05 IC12.14 | IC12.14 283.85,139.7 Q3.3 285.12,133.35 Q5.3 294,128.27 R49.2 299.09,124.46 R55.1 | IC12.14 274.96,143.51 274.96,128.27 Q1.3 271.14,124.16 267.97,124.16 | 267.97,124.16 257.48,124.16 D5.C | R56.1 R50.2 295.91,30.48 292.1,34.29 292.1,36.2 Q6.3 286.38,38.1 Q4.3 280.98,40.97 280.98,49.86 IC16.14 276.53,54.3 274.28,54.3 267.97,60.61 267.97,124.16
+15VDC  (via drill 0.35)
  Top 0.381: v266.7,232.79 267.84,231.65 267.84,217.55 268.99,217.55 C5.+
  Bottom 0.381: v266.7,232.79 264.03,235.46 264.03,257.18 261.75,259.46 R6.2
  Bottom 1.016: C5.+ 270.76,215.9 IC1.OUT 274.32,168.91 278.13,165.1 291.47,165.1 IC10.7 C37.1 302.89,146.05 309.25,146.05 IC11.8 | IC11.8 C33.1 | IC11.8 309.88,139.06 309.88,85.72 298.45,74.3 296.55,74.3 294,71.75 IC14.7 C50.1 302.89,53.34 309.25,53.34 IC15.8 C46.1
+22VDC
  Top 2.032: D1.C 300.36,253.37 | 300.36,253.37 300.36,239.4 | 300.36,239.4 D2.C 300.63,236.58 301.29,236.58 302.89,234.97 302.89,225.43 | IC2.IN 274.32,237.49 276.23,239.4 300.36,239.4 | IC3.IN 274.32,251.46 276.23,253.37 300.36,253.37 | C3.+ 302.89,220.34 302.89,225.43 | IC1.IN 274.32,223.52 276.23,225.43 302.89,225.43
-8VDC
  Top 0.762: R58.2 280.03,27.94 R52.1 271.78,33.66 271.78,67.94 273.86,70.03 276.23,70.03 | IC16.7 285.12,68.75 283.84,70.03 276.23,70.03 | 276.23,70.03 276.23,120.65 R51.1 | R51.1 R57.2 279.4,127.64 279.4,138.43 281.31,140.34 281.31,158.12 284.48,161.29 IC12.7 282.58,163.83 282.58,167.64 254.64,195.58 254.64,235.59 244.47,245.75 R10.2 | R15.1 257.18,129.54 264.8,121.92 R51.1
  Top 1.016: C8.- 267.72,259.33 262.89,264.16 248.92,264.16 R10.2
  Bottom 1.016: IC4.OUT 270.76,257.81 C8.-
-15VDC  (via drill 0.55)
  Top 1.016: C9.- 262.64,266.7 245.75,266.7 R11.2 | C47.1 IC15.4 295.58,67 290.81,67 283.85,73.97 C51.1 286.38,78.74 IC14.4 290.52,80.34 295.29,80.34 298.77,83.82 C44.1 304.8,87 304.8,99.69 300.36,104.14 C45.2 297.53,104.14 294.99,106.68 IC13.17 293.7,107.65 294.05,107.65 297.18,110.78 297.18,135.57 296.24,136.51 296.24,140.67 C34.1 IC11.4 296.85,158.44 290.81,158.44 285.12,164.14 C38.1 287.65,170.18 IC10.4 290.99,172.25 297.34,172.25 C31.1 300.05,178.1 300.05,184.16 300.66,184.77 300.66,191.15 299.09,192.73 C32.2 297.53,195.58 295.32,197.79 293.06,197.79 IC9.17 291.47,198.12 288.93,200.66 288.93,205.1 283.85,210.19 271.14,210.19 265.43,215.9 v265.43,240.66
  Bottom 1.016: IC5.OUT 270.76,271.78 C9.- 265.43,269.49 v265.43,240.66
/1DX0  (via drill 0.35)
  Top 0.381: v118.87,206.88 133.73,206.88 5C.2
  Bottom 0.381: 4C/4D.2 117.35,191.64 118.87,191.64 v118.87,206.88
/1DX1  (via drill 0.35)
  Top 0.381: v117.73,199.26 133.73,199.26 5C.5
  Bottom 0.381: v117.73,199.26 115.06,199.26 111.63,195.83 111.63,186.69 115.06,186.69 115.82,185.93 115.82,179.83 113.92,177.93 4C/4D.6
/1DX2
  Top 0.381: 4C/4D.10 127.64,186.69 135.64,186.69 139.45,190.5 142.88,190.5 143.64,191.26 143.64,196.6 141.73,196.6 5C.11
/1DX3  (via drill 0.35)
  Top 0.381: v109.73,210.69 132.59,210.69 132.97,211.07 139.06,211.07 v139.45,210.69
  Bottom 0.381: v109.73,210.69 109.73,185.17 111.25,185.17 113.54,182.88 4C/4D.4 | v139.45,210.69 139.45,206.5 141.35,204.6 5C.14
/1DX4
  Top 0.381: 5D.2 133.73,171.45 131.06,174.12 122.68,174.12 121.54,175.26 4C/4D.8
/1DX5
  Top 0.381: 4C/4D.12 121.16,185.17 118.11,182.12 118.11,165.35 132.21,165.35 133.73,163.83 5D.5
/1DX6  (via drill 0.35)
  Top 0.381: v115.82,157.35 116.21,156.97 130.68,156.97 132.97,154.69 v139.06,154.69
  Bottom 0.381: v115.82,157.35 115.82,154.31 113.92,152.4 4D/4E.2 | v139.06,154.69 139.45,155.07 139.45,159.26 141.35,161.16 5D.11
/1DX7  (via drill 0.35)
  Top 0.381: v139.45,176.4 v123.44,176.4
  Bottom 0.381: v123.44,176.4 123.44,166.88 111.63,166.88 110.49,165.74 110.49,145.54 113.54,142.49 4D/4E.6 | v139.45,176.4 139.45,171.07 5D.14
/1DX8
  Top 0.381: 5E.2 133.73,136.02 130.68,139.06 127.25,139.06 121.54,144.78 4D/4E.10
/1DX9
  Top 0.381: 5E.5 133.73,128.4 133.35,128.78 129.54,128.78 115.82,142.49 115.82,147.07 113.92,147.07 4D/4E.4
/1DX10
  Top 0.381: 5E.11 141.35,125.73 137.54,129.54 129.92,129.54 121.54,137.92 121.54,139.45 4D/4E.8
/1DX11
  Top 0.381: 4D/4E.12 121.54,149.73 121.92,149.35 128.02,149.35 128.78,148.59 128.78,143.64 128.4,143.64 127.64,142.88 127.64,139.83 135.25,139.83 141.73,133.35 5E.14
/1DY0  (via drill 0.35)
  Top 0.381: 4F/4G.2 121.92,89.53 v131.83,89.53
  Bottom 0.381: v131.83,89.53 131.83,98.3 133.73,100.2 5F.2
/1DY1
  Top 0.381: 4F/4G.6 113.92,71.25 116.97,71.25 119.25,73.53 119.25,80.01 130.3,80.01 134.11,83.82 135.25,83.82 136.02,84.58 136.02,92.58 134.11,92.58 5F.5
/1DY2
  Top 0.381: 4F/4G.10 125.35,77.72 131.06,77.72 139.45,86.11 139.45,89.92 141.35,89.92 5F.11
/1DY3  (via drill 0.35)
  Top 0.381: v118.49,89.92 v111.63,89.92 | v118.49,108.2 137.16,108.2 137.54,107.82 v139.45,107.82
  Bottom 0.381: v111.63,89.92 111.63,78.11 113.54,76.2 4F/4G.4 | v118.49,108.2 v118.49,89.92 | v139.45,107.82 139.45,99.82 141.35,97.92 5F.14
/1DY4
  Top 0.381: 5G.2 133.73,64.77 131.83,66.67 123.44,66.67 121.54,68.58 4F/4G.8
/1DY5  (via drill 0.35)
  Top 0.381: v120.4,57.15 5G.5
  Bottom 0.381: v120.4,57.15 120.4,67.06 119.25,68.2 119.25,76.58 121.16,78.49 4F/4G.12
/1DY6
  Top 0.381: 4G/4H.2 113.92,45.72 115.82,47.62 115.82,51.44 126.87,51.44 127.25,51.05 130.3,51.05 132.59,53.34 139.06,53.34 140.21,54.48 141.35,54.48 5G.11
/1DY7  (via drill 0.35)
  Top 0.381: v119.25,58.67 121.54,60.96 139.06,60.96 140.21,62.1 141.35,62.1 5G.14
  Bottom 0.381: 4G/4H.6 117.35,39.24 117.35,43.05 119.25,44.96 v119.25,58.67
/1DY8
  Top 0.381: 4G/4H.4 113.54,40.39 110.87,37.72 110.87,30.48 123.83,30.48 124.21,30.1 128.4,30.1 129.16,29.34 133.73,29.34 5H.2
/1DY9  (via drill 0.35)
  Top 0.381: v121.54,21.72 133.73,21.72 5H.5
  Bottom 0.381: v121.54,21.72 121.54,32.77 4G/4H.8
/1DY10  (via drill 0.35)
  Top 0.381: v139.45,40.01 138.3,41.15 129.92,41.15 128.02,43.05 121.54,43.05 4G/4H.12
  Bottom 0.381: v139.45,40.01 139.45,30.48 142.88,30.48 143.64,29.72 143.64,20.96 141.73,19.05 5H.11
/1DY11
  Top 0.381: 5H.14 141.73,26.67 143.64,28.58 143.64,35.43 124.21,35.43 121.54,38.1 4G/4H.10
/COUNT  (via drill 0.35)
  Top 0.381: v118.49,224.79 4B.11 v96.01,224.79 | v118.49,236.22 128.78,236.22 132.59,232.41 138.68,232.41 | 138.68,232.41 139.06,232.41 140.21,233.55 141.35,233.55 5B.10 | v62.48,219.84 66.29,216.03 v87.63,216.03 | v148.97,268.99 154.31,268.99 6A.5 | v148.97,225.93 148.59,226.31 139.06,226.31 138.68,226.69 138.68,232.41 | 8D/8E.13 v198.12,148.59 | v148.97,219.46 149.35,219.84 199.64,219.84 v200.03,219.46
  Bottom 0.381: v118.49,236.22 v118.49,224.79 | v62.48,219.84 62.48,234.31 60.58,236.22 1B.11 | v87.63,216.03 88.77,217.17 96.01,217.17 v96.01,224.79 | v148.97,268.99 v148.97,225.93 v148.97,219.46 | 8G/8H.10 202.69,34.29 202.69,36.58 8G/8H.11 204.6,38.86 204.6,40.01 202.69,41.91 8G/8H.13 202.31,41.91 200.41,43.81 200.41,49.91 204.6,54.1 204.6,75.44 8F/8G.13 199.64,80.39 199.64,89.15 200.03,89.53 200.03,97.92 204.6,102.49 204.6,145.54 | 8D/8E.10 202.69,140.97 202.69,143.26 8D/8E.11 204.6,145.54 | 204.6,145.54 204.6,146.69 202.69,148.59 8D/8E.13 | v198.12,148.59 198.12,179.83 202.31,184.02 8C/8D.13 202.69,184.4 204.6,186.31 204.6,190.5 201.17,190.5 200.41,191.26 200.41,207.26 200.03,207.65 v200.03,219.46
/DX=0  (via drill 0.35)
  Top 0.381: v58.29,283.08 94.87,283.08 95.25,283.46 104.01,283.46 104.39,283.08 105.16,283.08 105.54,283.46 124.59,283.46 124.97,283.08 v139.45,283.08 | v139.45,278.13 155.45,278.13 158.5,275.08 158.5,259.84 v174.5,259.84
  Bottom 0.381: v58.29,283.08 58.29,276.23 60.2,274.32 1A.12 | v139.45,278.13 v139.45,283.08 | v174.5,259.84 174.5,243.84 7B.1
/DY=0
  Top 0.381: 6A.12 166.88,279.27 174.5,279.27 7A.1
/FRAMECOMPLETE  (via drill 0.35)
  Top 0.381: v152.78,254.13 135.25,254.13 134.87,254.51 117.35,254.51 116.21,255.65 115.44,255.65 115.06,255.27 102.11,255.27 101.73,255.65 78.87,255.65 64.01,270.51 54.1,270.51 52.96,271.65 1A.4
  Bottom 0.381: v152.78,254.13 152.4,253.75 152.4,238.12 B6.4
/HALTROTATE  (via drill 0.35)
  Top 0.381: v138.3,219.46 137.92,219.84 133.73,219.84 133.35,219.46 105.54,219.46 105.16,219.07 100.97,219.07 100.2,219.84 v97.92,219.84 | v87.63,214.88 76.2,214.88 75.82,215.27 55.63,215.27 v55.25,215.65
  Bottom 0.381: 54.86,245.75 52.96,243.84 1B.1 | 54.86,245.75 54.86,277.37 52.96,279.27 1A.1 | v138.3,219.46 138.3,228.98 139.45,230.12 139.45,239.27 141.35,241.17 5B.13 | v97.92,219.84 97.54,219.46 97.54,207.65 95.63,205.74 89.54,205.74 89.54,212.98 v87.63,214.88 | v55.25,215.65 55.25,245.36 54.86,245.75
/INHIBITX  (via drill 0.35)
  Top 0.381: 7A.10 188.59,262.89 v192.79,262.89 221.74,262.89 222.88,264.03 9A.8
  Bottom 0.381: v192.79,262.89 192.79,240.79 194.69,238.89 8B.3
/INHIBITY  (via drill 0.35)
  Top 0.381: 7B.10 186.31,237.74 188.98,237.74 195.07,243.84 | v217.17,246.51 216.79,246.13 197.36,246.13 195.07,243.84 | 195.07,243.84 8B.1
  Bottom 0.381: v217.17,246.51 217.17,275.84 216.03,275.84 215.26,276.61 9A.2
/LDROT  (via drill 0.35)
  Top 0.381: v167.26,224.79 135.25,224.79 131.44,228.6 123.83,228.6 122.68,229.74 110.11,229.74 4B.9 | v167.26,271.65 161.93,271.65 6A.11
  Bottom 0.381: v167.26,271.65 v167.26,224.79
/LDX2  (via drill 0.35)
  Top 0.381: v99.06,244.98 99.44,245.36 109.73,245.36 4B.3
  Bottom 0.381: v99.06,244.98 99.06,233.17 100.97,231.27 3B.9
/LDXY1  (via drill 0.35)
  Top 0.381: v107.44,232.41 99.82,232.41 99.06,233.17 93.73,233.17 93.34,233.55 3B.5
  Bottom 0.381: v107.44,232.41 107.82,232.79 107.82,235.46 108.59,236.22 112.01,236.22 112.01,248.03 4B.1
/LDY2
  Top 0.381: 4B.5 99.82,240.03 98.68,238.89 93.34,238.89 3B.3
/LDZ  (via drill 0.35)
  Top 0.381: v122.68,235.08 110.11,235.08 4B.7 | v128.4,280.8 155.45,280.8 159.26,276.99 159.26,266.7 6A.9
  Bottom 0.381: v122.68,235.08 123.06,235.46 123.06,243.08 123.83,243.84 128.4,243.84 v128.4,280.8
/ROTATE  (via drill 0.35)
  Top 0.381: 4B.10 111.25,225.93 118.87,225.93 123.83,220.98 132.59,220.98 133.35,221.74 v139.45,221.74 | v156.59,265.94 156.59,263.27 v156.21,263.27 | v152.02,232.79 150.5,231.27 141.73,231.27 5B.9
  Bottom 0.381: v139.45,221.74 139.45,228.98 5B.9 | v156.59,265.94 156.59,276.99 154.31,279.27 6A.1 | v156.21,263.27 151.64,258.7 151.64,233.17 v152.02,232.79
/SUBTRACT  (via drill 0.35)
  Top 0.381: v114.3,252.22 121.16,252.22 122.68,253.75 134.49,253.75 135.25,252.98 v144.02,252.98 | 6A.3 v144.02,274.32
  Bottom 0.381: v114.3,252.22 114.3,236.6 110.11,232.41 4B.8 | v144.02,274.32 v144.02,252.98
/TTLINVX  (via drill 0.35)
  Top 0.381: R47.1 293.37,120.02 v277.37,120.02 | v262.89,107.82 v275.08,107.82 | v262.89,7.24 259.46,3.81 29.72,3.81 v25.65,7.87 | v25.65,116.2 5.08,116.2 P1.19
  Bottom 0.381: v277.37,120.02 275.08,117.73 v275.08,107.82 | v262.89,7.24 v262.89,107.82 | v25.65,116.2 v25.65,7.87
/TTLINVY  (via drill 0.35)
  Top 0.381: v296.8,7.24 292.61,3.05 28.32,3.05 24.51,6.86 v24.51,9.02 | v24.51,114.3 v5.08,114.3
  Bottom 0.381: v296.8,7.24 296.8,24 R48.1 | v24.51,114.3 v24.51,9.02 | v5.08,114.3 5.08,116.2 P1.W
/VRAMPC1
  Top 0.381: 3B.11 111.25,236.22 114.3,239.27 114.3,247.65 4B.2
/VRAMPC2
  Top 0.381: 3B.13 100.97,241.55 101.73,242.32 109.73,242.32 4B.4
/VRAMPC3  (via drill 0.35)
  Top 0.381: 4B.6 112.01,239.65 v113.16,239.65 | v113.16,251.46 104.01,251.46 96.39,243.84 3B.1
  Bottom 0.381: v113.16,251.46 v113.16,239.65
/XCUR0  (via drill 0.35)
  Top 0.381: v98.68,203.84 98.68,211.07 95.25,211.07 86.49,219.84 v85.73,219.84 | v85.73,240.03 74.3,240.03 2B.2
  Bottom 0.381: v98.68,203.84 98.68,199.26 100.97,196.98 3C.11 | v85.73,240.03 v85.73,219.84
/XCUR1  (via drill 0.35)
  Top 0.381: v45.72,227.46 46.1,227.08 53.72,227.08 59.06,232.41 61.72,232.41 62.1,232.79 69.34,232.79 72.77,236.22 2B.4 | v45.72,186.31 91.44,186.31 v91.82,185.93
  Bottom 0.381: v45.72,186.31 v45.72,227.46 | v91.82,185.93 91.44,186.31 91.44,192.41 3C.7
/XCUR2
  Top 0.381: 3C.4 87.25,201.93 87.25,209.55 88.01,210.31 88.77,210.31 88.77,216.41 86.87,218.31 85.73,218.31 73.15,230.89 2B.6
/XCUR3
  Top 0.381: 3C.16 100.97,209.93 99.06,211.84 95.63,211.84 86.49,220.98 84.2,220.98 80.77,224.41 80.77,228.6 2B.8
/XCUR4  (via drill 0.35)
  Top 0.381: v76.58,225.93 75.82,225.17 v57.53,225.17 | v57.15,163.83 74.3,163.83 78.49,159.64 78.49,155.83 88.01,155.83 91.44,152.4 v99.06,152.4
  Bottom 0.381: v76.58,225.93 76.58,233.55 80.39,233.55 2B.10 | v57.53,225.17 57.53,177.93 57.15,177.55 v57.15,163.83 | v99.06,152.4 99.06,159.26 100.97,161.16 3D.11
/XCUR5  (via drill 0.35)
  Top 0.381: v97.16,240.03 92.2,240.03 91.06,238.89 80.77,238.89 2B.12 | v96.39,208.03 95.25,206.88 v95.25,203.45 | v98.3,181.74 v90.68,181.74 | v98.3,167.64 98.3,161.93 95.25,158.88 93.34,158.88 3D.7
  Bottom 0.381: v97.16,240.03 97.16,220.6 96.77,220.22 96.77,208.41 v96.39,208.03 | v95.25,203.45 95.25,198.88 94.49,198.12 90.68,198.12 v90.68,181.74 | v98.3,181.74 97.92,181.36 97.92,168.02 v98.3,167.64
/XCUR6  (via drill 0.35)
  Top 0.381: v89.54,168.78 86.87,171.45 74.3,171.45 2D.2
  Bottom 0.381: v89.54,168.78 89.54,166.5 93.34,166.5 3D.4
/XCUR7  (via drill 0.35)
  Top 0.381: v100.97,182.88 v70.87,182.88
  Bottom 0.381: 2D.4 70.87,167.26 v70.87,182.88 | 3D.16 v100.97,182.88
/XCUR8  (via drill 0.35)
  Top 0.381: v107.44,125.73 3E.11 | v107.44,138.3 105.92,139.83 89.92,139.83 89.54,139.45 88.77,139.45 88.01,140.21 88.01,146.69 88.77,147.45 88.77,148.97 84.2,148.97 73.15,160.02 2D.6
  Bottom 0.381: v107.44,138.3 v107.44,125.73
/XCUR9  (via drill 0.35)
  Top 0.381: v89.54,157.35 80.77,157.35 2D.8
  Bottom 0.381: v89.54,157.35 89.92,156.97 89.92,141.35 90.68,140.59 90.68,131.06 92.2,129.54 95.25,129.54 95.25,124.97 93.34,123.06 3E.7
/XCUR10  (via drill 0.35)
  Top 0.381: v90.3,162.31 80.77,162.31 2D.10
  Bottom 0.381: v90.3,162.31 90.68,161.93 90.68,141.73 91.44,140.97 91.44,132.59 93.34,130.68 3E.4
/XCUR11  (via drill 0.35)
  Top 0.381: v90.68,167.64 2D.12 | v95.63,138.68 100.97,138.68 3E.16
  Bottom 0.381: v90.68,167.64 95.63,167.64 v95.63,138.68
/YCUR0
  Top 0.381: 3F.11 100.97,89.92 100.2,89.15 99.82,89.15 94.49,83.82 59.06,83.82 58.29,84.58 58.29,91.44 65.15,91.44 72.77,99.06 2F.2
/YCUR1
  Top 0.381: 3F.7 71.63,87.63 70.87,88.39 70.87,93.73 72.77,93.73 2F.4
/YCUR2
  Top 0.381: 3F.4 77.34,95.25 77.34,93.34 73.15,89.15 2F.6
/YCUR3  (via drill 0.35)
  Top 0.381: v91.44,86.49 80.77,86.49 2F.8
  Bottom 0.381: v91.44,86.49 91.44,90.68 92.2,91.44 96.01,91.44 96.01,97.92 3F.16
/YCUR4  (via drill 0.35)
  Top 0.381: v82.68,77.72 88.01,72.39 96.39,72.39 99.82,68.96 110.49,68.96 110.49,62.48 103.63,55.63 101.73,55.63 100.97,54.86 3G.11
  Bottom 0.381: v82.68,77.72 82.68,89.53 80.77,91.44 2F.10
/YCUR5  (via drill 0.35)
  Top 0.381: v88.39,90.68 v83.06,90.68 | v91.44,74.68 v88.39,77.72
  Bottom 0.381: 2F.12 83.06,94.11 v83.06,90.68 | v88.39,77.72 v88.39,90.68 | v91.44,74.68 91.44,61.72 92.2,60.96 96.01,60.96 96.01,53.72 94.49,52.2 93.34,52.2 3G.7
/YCUR6  (via drill 0.35)
  Top 0.381: v89.54,32.77 77.72,32.77 73.15,28.19 2H.2
  Bottom 0.381: v89.54,32.77 89.54,50.67 92.2,53.34 94.49,53.34 95.25,54.1 95.25,57.91 93.34,59.82 3G.4
/YCUR7  (via drill 0.35)
  Top 0.381: v97.92,38.1 v70.87,38.1
  Bottom 0.381: v70.87,38.1 70.87,24.77 72.77,22.86 2H.4 | v97.92,38.1 98.3,38.48 98.3,64.77 100.97,67.44 3G.16
/YCUR8  (via drill 0.35)
  Top 0.381: v97.92,12.19 78.49,12.19 73.15,17.53 2H.6
  Bottom 0.381: v97.92,12.19 98.3,12.57 98.3,16.38 3H.11
/YCUR9
  Top 0.381: 2H.8 80.77,15.24 81.92,16.38 93.34,16.38 3H.7
/YCUR10
  Top 0.381: 2H.10 80.77,20.57 84.2,24 93.34,24 3H.4
/YCUR11  (via drill 0.35)
  Top 0.381: v82.68,28.96 84.2,30.48 98.68,30.48 99.82,31.62 100.97,31.62 3H.16
  Bottom 0.381: 2H.12 82.68,27.43 v82.68,28.96
A  (via drill 0.35)
  Top 0.381: v300.23,78.11 308.99,69.34 308.99,58.67 313.56,58.67 314.33,57.91 314.33,48.01 309.75,48.01 308.23,49.53 IC15.6
  Bottom 0.381: IC13.18 292.99,109.35 299.09,109.35 R45.2 R41.1 300.61,105.16 300.61,89.92 300.23,89.53 v300.23,78.11 | 302.89,43.05 301.75,44.2 R37.2 | C43.2 302.89,43.05 | 302.89,43.05 302.89,44.58 307.85,49.53 IC15.6
B  (via drill 0.35)
  Top 0.381: IC9.18 292.99,200.79 299.09,200.79 R34.2 | R26.2 302.89,137.16 IC11.6 307.85,142.49 307.85,146.3 v306.71,147.45
  Bottom 0.381: R34.2 R30.1 306.71,190.5 v306.71,147.45 | C30.2 302.89,136.02 301.75,137.16 R26.2
BEAMOFF
  Bottom 0.381: 9A.12 224.79,272.41 224.79,263.65 219.46,258.32 219.46,234.7 216.03,234.7 215.26,233.93 9B.5
BEAMON  (via drill 0.35)
  Top 0.381: v74.68,255.27 75.06,254.89 101.35,254.89 101.73,254.51 v115.82,254.51 | v197.74,211.84 v117.35,211.84 | v225.17,245.36 198.88,245.36 195.07,241.55 8B.2
  Bottom 0.381: 8B.2 196.98,239.27 196.98,238.12 195.07,236.22 8B.4 194.69,236.22 192.79,234.31 192.79,232.41 196.22,232.41 197.74,230.89 v197.74,211.84 | v74.68,255.27 75.06,255.65 75.06,272.41 73.15,274.32 2A.3 | v115.82,254.51 117.35,254.51 v117.35,211.84 | v225.17,245.36 225.55,245.75 225.55,275.84 223.65,275.84 222.88,276.61 9A.13
BTTMPLANE
  pour Bottom (isolate 0.381): 229.24,290.83 316.23,290.83 328.93,278.13 328.93,277.5 328.93,10.16 320.68,1.91 313.06,1.91 254,1.91 254,225.43 229.24,250.19
COUNT  (via drill 0.35)
  Top 0.381: v188.59,238.89 182.5,238.89 7B.12 | v160.02,252.6 v188.59,252.6 | v188.59,272.8 v184.4,272.8
  Bottom 0.381: 159.64,252.6 159.64,261.37 6A.6 | 159.64,252.6 159.64,234.7 161.16,234.7 161.93,233.93 B6.10 | v188.59,238.89 v188.59,252.6 v188.59,272.8 | 159.64,252.6 v160.02,252.6 | 7A.13 184.4,274.7 v184.4,272.8
DACX0  (via drill 0.35)
  Top 0.381: v237.36,205.74 221.74,205.74 220.98,204.98 215.65,204.98 215.26,204.6 9C.3 | v237.36,195.45 237.74,195.07 238.12,195.07 239.65,193.55 v239.65,191.26 | IC9.12 291.47,186.69 282.32,186.69 281.94,187.07 266.32,187.07 260.6,192.79 v259.08,192.79 | v255.65,192.79 254.13,194.31 10C.10
  Bottom 0.381: v237.36,205.74 237.74,205.36 237.74,195.83 v237.36,195.45 | v239.65,191.26 242.7,194.31 10C.10 | v255.65,192.79 v259.08,192.79
DACX1  (via drill 0.35)
  Top 0.381: v216.79,216.79 217.17,217.17 249.56,217.17 251.46,215.27 251.46,199.64 243.46,199.64 10C.12 | v271.27,180.59 290.32,180.59 292.61,182.88 IC9.11 | v245.36,178.69 v269.75,178.69
  Bottom 0.381: v216.79,216.79 217.17,216.41 217.17,208.03 216.03,208.03 215.26,207.26 9C.2 | v271.27,180.59 269.75,179.07 v269.75,178.69 | v245.36,178.69 245.36,197.36 243.46,199.26 10C.12
DACX2  (via drill 0.35)
  Top 0.381: v220.6,201.17 216.79,197.36 215.65,197.36 215.26,196.98 9C.6 | v221.74,211.07 236.6,211.07 241.17,206.5 241.17,201.93 | 10C.13 241.17,201.93 | v261.37,190.5 265.56,186.31 281.56,186.31 284.99,182.88 IC9.10 | v257.94,190.5 241.94,190.5 240.41,192.02 240.41,201.93 241.17,201.93
  Bottom 0.381: v220.6,201.17 220.98,201.55 220.98,210.31 v221.74,211.07 | v257.94,190.5 v261.37,190.5
DACX3  (via drill 0.35)
  Top 0.381: IC9.9 287.27,183.26 287.27,181.36 272.03,181.36 271.65,181.74 v270.13,181.74 | v250.32,179.83 v268.61,179.83 | v250.32,206.88 243.46,206.88 10C.15 | v209.93,194.31 9C.7 | v209.93,219.46 210.31,219.84 216.41,219.84 217.55,220.98 v250.7,220.98
  Bottom 0.381: v270.13,181.74 268.61,180.21 v268.61,179.83 | v250.32,179.83 v250.32,206.88 250.7,207.26 v250.7,220.98 | v209.93,219.46 v209.93,194.31
DACX4  (via drill 0.35)
  Top 0.381: v272.8,158.88 v250.7,158.88 243.46,158.88 10D.10 | v272.8,188.21 284.99,188.21 IC9.8 | v216.41,176.78 213.36,176.78 213.36,170.69 214.12,169.93 214.5,169.93 215.26,169.16 9D.3 | v248.41,219.84 v217.93,219.84
  Bottom 0.381: v272.8,188.21 v272.8,158.88 | v216.41,176.78 217.93,178.31 v217.93,219.84 | v248.41,219.84 248.41,167.64 250.7,165.35 v250.7,158.88
DACX5  (via drill 0.35)
  Top 0.381: 9D.2 219.07,167.64 v230.5,167.64 | v250.7,106.68 v229.36,106.68 | 10D.12 v249.56,163.83 273.94,163.83 v277.75,167.64
  Bottom 0.381: v230.5,167.64 230.5,110.49 229.36,109.35 v229.36,106.68 | v250.7,106.68 250.7,157.35 249.56,158.5 v249.56,163.83 | v277.75,167.64 277.75,171.83 277.37,172.21 277.37,182.88 284.99,190.5 IC9.7
DACX6  (via drill 0.35)
  Top 0.381: v209.93,161.16 215.26,161.16 9D.6 | v209.93,116.59 210.31,116.97 226.31,116.97 227.84,115.44 237.36,115.44 v237.74,115.82 | v248.41,109.35 v237.74,109.35 | 10D.13 243.46,166.12 v248.41,166.12 v263.65,166.12 | v263.65,192.79 284.99,192.79 IC9.6
  Bottom 0.381: v209.93,161.16 210.31,160.78 210.31,116.97 v209.93,116.59 | v237.74,109.35 v237.74,115.82 | v248.41,166.12 v248.41,109.35 | v263.65,166.12 v263.65,192.79
DACX7  (via drill 0.35)
  Top 0.381: v219.07,158.88 215.26,158.88 9D.7 | v219.07,216.03 249.17,216.03 v249.56,215.65 | 10D.15 v249.56,171.45 v276.61,171.45
  Bottom 0.381: v219.07,216.03 v219.07,158.88 | v249.56,215.65 249.17,215.27 249.17,171.83 v249.56,171.45 | IC9.5 276.61,187.07 v276.61,171.45
DACX8  (via drill 0.35)
  Top 0.381: 9E.3 221.74,139.83 v229.36,139.83 | v228.22,107.82 248.41,107.82 250.7,110.11 250.7,123.06 | 250.7,123.06 243.46,123.06 10E.10 | v251.84,169.55 v275.84,169.55 | 250.7,123.06 v251.84,123.06
  Bottom 0.381: v229.36,139.83 229.36,110.49 228.22,109.35 v228.22,107.82 | v275.84,169.55 275.46,169.93 275.46,188.59 284.99,198.12 IC9.4 | v251.84,123.06 v251.84,169.55
DACX9  (via drill 0.35)
  Top 0.381: v209.17,135.64 215.26,135.64 9E.2 | v208.79,111.63 245.75,111.63 246.51,112.4 246.51,121.92 241.94,121.92 241.17,122.68 241.17,128.02 243.08,128.02 10E.12 243.46,128.4 248.41,133.35 v262.13,133.35 | v262.51,200.41 284.99,200.41 IC9.3
  Bottom 0.381: v209.17,135.64 209.17,117.35 208.79,116.97 v208.79,111.63 | v262.51,200.41 262.51,136.78 262.13,136.4 v262.13,133.35
DACX10
  Top 0.381: 9E.6 217.17,127.64 219.84,127.64 221.74,129.54 241.94,129.54 10E.13
DACX11  (via drill 0.35)
  Top 0.381: v237.74,83.06 v224.79,83.06 | v253.75,91.44 v238.89,91.44 | v256.41,132.21 262.51,132.21 263.27,132.97 263.27,134.49 244.6,134.49 10E.15
  Bottom 0.381: v224.79,83.06 224.79,99.06 221.74,99.06 220.98,99.82 220.98,100.97 217.55,104.39 217.55,120.78 215.26,123.06 9E.7 | v237.74,83.06 238.89,83.06 v238.89,91.44 | v253.75,91.44 253.75,126.87 256.41,129.54 v256.41,132.21
DACY0  (via drill 0.35)
  Top 0.381: v273.94,87.63 10F.10 | v277.37,95.25 291.47,95.25 IC13.12 | v212.98,115.82 213.36,115.44 226.69,115.44 227.46,114.68 238.51,114.68 v238.89,115.06
  Bottom 0.381: v273.94,87.63 273.94,92.96 276.23,95.25 v277.37,95.25 | v212.98,115.82 212.6,115.44 212.6,100.58 215.26,97.92 9F.3 | v238.89,115.06 238.89,92.96 241.17,90.68 241.17,89.53 243.08,87.63 10F.10
DACY1  (via drill 0.35)
  Top 0.381: v213.74,108.2 226.31,108.2 230.12,104.39 236.6,104.39 241.17,99.82 241.17,92.96 243.08,92.96 10F.12 243.46,92.58 v275.08,92.58 | v277.37,89.92 291.08,89.92 292.61,91.44 IC13.11
  Bottom 0.381: v213.74,108.2 213.36,107.82 213.36,101.35 214.5,101.35 215.26,100.58 9F.2 | v277.37,89.92 275.08,92.2 v275.08,92.58
DACY2  (via drill 0.35)
  Top 0.381: v237.74,81.91 v216.79,81.91 | v240.03,83.82 v248.41,83.82 v275.08,83.82 | 10F.13 v248.41,95.25
  Bottom 0.381: v216.79,81.91 217.17,82.3 217.17,89.15 216.03,89.15 215.26,89.92 9F.6 | v237.74,81.91 240.03,81.91 v240.03,83.82 | v248.41,95.25 v248.41,83.82 | v275.08,83.82 277.37,83.82 284.99,91.44 IC13.10
DACY3  (via drill 0.35)
  Top 0.381: v207.65,87.63 9F.7 | v207.65,117.73 240.79,117.73 v241.17,117.35 | v275.08,100.2 243.46,100.2 10F.15
  Bottom 0.381: v207.65,117.73 v207.65,87.63 | v241.17,117.35 241.17,102.49 243.08,100.58 10F.15 | IC13.9 279.65,99.44 275.08,99.44 v275.08,100.2
DACY4  (via drill 0.35)
  Top 0.381: v213.36,51.05 213.36,48.01 v238.51,48.01 | v270.51,60.2 262.51,52.2 243.46,52.2 10G.10
  Bottom 0.381: v213.36,51.05 213.36,60.2 215.26,62.1 9G.3 | v238.51,48.01 242.32,51.82 243.08,51.82 10G.10 | v270.51,60.2 271.65,61.34 271.65,101.35 275.46,101.35 276.23,100.58 276.23,100.2 280.03,100.2 283.46,96.77 284.99,96.77 IC13.8
DACY5  (via drill 0.35)
  Top 0.381: 9G.2 219.07,68.58 227.84,68.58 230.12,66.29 v233.55,66.29 | v275.08,102.49 273.94,101.35 v245.36,101.35
  Bottom 0.381: v233.55,66.29 233.55,67.82 235.84,70.1 240.41,70.1 | 240.41,70.1 241.17,70.1 241.17,59.05 243.08,57.15 10G.12 | IC13.7 282.32,99.06 280.42,100.97 276.99,100.97 275.46,102.49 v275.08,102.49 | v245.36,101.35 245.36,81.53 240.41,76.58 240.41,70.1
DACY6  (via drill 0.35)
  Top 0.381: v237.74,53.34 221.74,53.34 220.98,54.1 215.65,54.1 215.26,54.48 9G.6 | v237.74,59.44 243.08,59.44 10G.13 243.46,59.82 268.61,59.82 v270.51,61.72
  Bottom 0.381: v237.74,59.44 v237.74,53.34 | v270.51,61.72 270.51,103.63 275.46,103.63 277.37,101.73 284.99,101.73 IC13.6
DACY7  (via drill 0.35)
  Top 0.381: v237.36,46.86 212.22,46.86 212.22,51.44 212.98,52.2 215.26,52.2 9G.7 | 10G.15 v269.37,64.77
  Bottom 0.381: v237.36,46.86 237.36,45.34 238.12,44.58 245.36,44.58 245.36,62.87 243.46,64.77 10G.15 | v269.37,64.77 269.37,104.39 284.99,104.39 IC13.5
DACY8  (via drill 0.35)
  Top 0.381: v237.36,30.48 219.07,30.48 9H.3 | v250.7,105.54 v275.08,105.54 | v250.7,16.76 243.46,16.76 10H.10
  Bottom 0.381: v237.36,30.48 237.74,30.1 237.74,22.1 243.08,16.76 10H.10 | IC13.4 283.85,106.68 282.7,105.54 v275.08,105.54 | v250.7,16.76 v250.7,105.54
DACY9  (via drill 0.35)
  Top 0.381: v237.74,33.15 219.07,33.15 215.26,29.34 9H.2 | v251.84,106.68 v275.08,106.68 | v251.84,21.72 243.46,21.72 10H.12
  Bottom 0.381: 10H.12 239.65,25.15 239.65,31.62 238.12,33.15 v237.74,33.15 | v275.08,106.68 282.7,106.68 284.99,108.97 IC13.3 | v251.84,21.72 v251.84,106.68
DACY10
  Top 0.381: 9H.6 219.07,22.86 240.79,22.86 241.94,24 243.08,24 10H.13
DACY11  (via drill 0.35)
  Top 0.381: v246.13,9.91 v217.17,9.91
  Bottom 0.381: v217.17,9.91 217.17,14.48 215.26,16.38 9H.7 | v246.13,9.91 246.13,26.29 10H.15
DX0
  Top 0.381: 7C.2 140.21,205.74 139.06,204.6 136.78,204.6 134.11,201.93 5C.4
DX1  (via drill 0.35)
  Top 0.381: v137.54,194.31 5C.7 | v169.55,187.07 v137.54,187.07 | v169.55,203.07 174.5,203.07 7C.3
  Bottom 0.381: v137.54,187.07 v137.54,194.31 | v169.55,203.07 v169.55,187.07
DX2  (via drill 0.35)
  Top 0.381: v176.78,183.64 v141.73,183.64
  Bottom 0.381: v141.73,183.64 141.73,191.64 5C.9 | v176.78,183.64 176.78,198.5 7C.4
DX3
  Top 0.381: 5C.12 142.11,198.88 152.4,198.88 153.16,198.12 7C.5
DX4  (via drill 0.35)
  Top 0.381: v136.4,174.12 139.06,174.12 141.73,176.78 v172.59,176.78
  Bottom 0.381: 5D.4 136.4,168.78 v136.4,174.12 | v172.59,176.78 172.59,172.21 7D.2
DX5
  Top 0.381: 7D.3 176.78,167.64 176.78,164.59 176.02,163.83 173.36,163.83 169.55,160.02 160.78,160.02 155.45,154.69 140.59,154.69 139.45,155.83 136.78,155.83 134.11,158.5 5D.7
DX6
  Top 0.381: 5D.9 141.73,156.21 153.16,167.64 172.21,167.64 174.5,165.35 7D.4
DX7  (via drill 0.35)
  Top 0.381: v177.17,176.02 176.78,175.64 153.54,175.64 151.26,173.36 151.26,166.88 144.78,166.88 141.73,163.83 5D.12
  Bottom 0.381: v177.17,176.02 177.17,164.97 174.88,162.69 7D.5
DX8  (via drill 0.35)
  Top 0.381: v131.83,144.02 172.97,144.02 173.74,143.26 173.74,138.68 172.59,137.54 172.59,134.87 174.5,134.87 7E.2
  Bottom 0.381: 5E.4 131.83,132.97 v131.83,144.02
DX9  (via drill 0.35)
